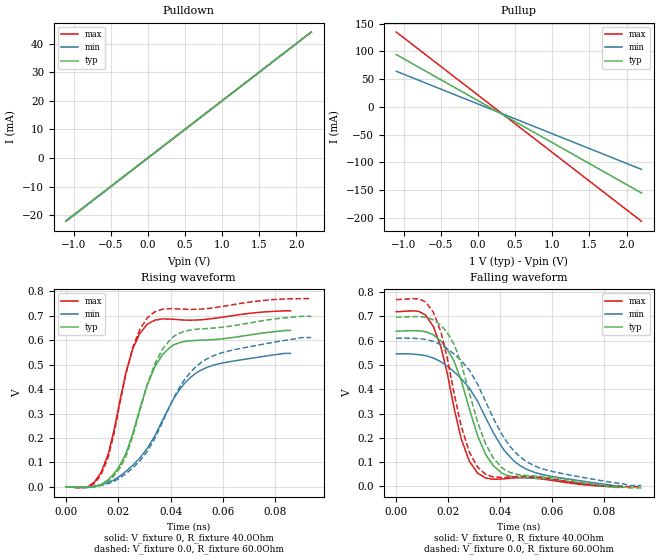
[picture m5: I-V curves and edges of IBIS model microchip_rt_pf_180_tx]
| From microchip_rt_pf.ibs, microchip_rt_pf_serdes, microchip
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|   MODEL microchip_rt_pf_180_tx
[Model] microchip_rt_pf_180_tx
Model_type   Output
Polarity   Non-Inverting
Enable   Active-High
Vmeas = 0.5
|   typ   min   max
C_comp   0.407p  0.407p  0.407p
[Voltage Range]   1.0  0.9  1.1
[Temperature Range]   60   100   0
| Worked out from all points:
|   slope of the pulldown table from 0 to 0.15 V, typ, clamps not added: 50.1 ohm
|   slope of the pullup table from 0 to 0.15 V, typ, clamps not added: 13.2 ohm
|   rising waveform, V_fixture 0, R_fixture 40.0Ohm: 20-80 % time 12.6ps typ, 19.1ps min, 9.64ps max; typ from 0 V to 0.64 V
|   rising waveform, V_fixture 0.0, R_fixture 60.0Ohm: 20-80 % time 13.3ps typ, 20ps min, 10.3ps max; typ from 0 V to 0.697 V
|   falling waveform, V_fixture 0, R_fixture 40.0Ohm: 20-80 % time 12.4ps typ, 19.3ps min, 9.67ps max; typ from 0.64 V to -0.004 V
|   falling waveform, V_fixture 0.0, R_fixture 60.0Ohm: 20-80 % time 13.2ps typ, 20.1ps min, 10.1ps max; typ from 0.697 V to -0.006 V
[Pullup]
|   X   TYP   MIN   MAX
-1.1V     94.44mA    64.32mA    135mA
1.01V     -65.12mA   -48.81mA   -83.11mA
1.089V    -71.06mA   -53.03mA   -91.23mA
2.2V      -155.1mA   -112.6mA   -206.1mA
[Pulldown]
|   X   TYP   MIN   MAX
-1.1V     -21.87mA   -22.07mA   -21.96mA
1.01V     20.25mA    20.18mA    20.22mA
1.066V    21.37mA    21.3mA     21.34mA
2.2V      44mA       44mA       44mA
[Ramp]
R_load = 50.0Ohm
|   typ   min   max
dV/dt_r   3.84E-1V/1.26E-2ns   3.27E-1V/1.91E-2ns   4.32E-1V/9.44E-3ns
dV/dt_f   3.86E-1V/1.24E-2ns   3.26E-1V/1.91E-2ns   4.33E-1V/9.31E-3ns
[Rising Waveform]
V_fixture   = 0
V_fixture_min = 0
V_fixture_max = 0
R_fixture   = 40.0Ohm
|   Time   V(typ)   V(min)   V(max)
0s        0V         0V         0V
8.626ps   -1.84mV    992.9uV    2.54mV
13.37ps   9.403mV    8.849mV    59.23mV
16.09ps   29.13mV    18.22mV    133.4mV
22.82ps   134.6mV    63.07mV    465.2mV
25.49ps   218.2mV    88.68mV    564.8mV
31.02ps   417.2mV    157.2mV    665mV
39.89ps   572mV      336.7mV    686mV
49.78ps   598.8mV    466.4mV    682.1mV
85.75ps   639.5mV    545.8mV    719.8mV
[Rising Waveform]
V_fixture   = 0.0
V_fixture_min = 0.0
V_fixture_max = 0.0
R_fixture   = 60.0Ohm
|   Time   V(typ)   V(min)   V(max)
0s        0V         0V         0V
8.626ps   -2.469mV   42.16uV    149.9uV
13.37ps   6.198mV    6.082mV    49.96mV
16.09ps   23.12mV    13.86mV    121.3mV
20.45ps   75.4mV     35.54mV    335.6mV
25.49ps   207.4mV    77.59mV    570.5mV
33.92ps   503.4mV    198.4mV    716mV
41.15ps   615.1mV    363.8mV    728.6mV
51.86ps   646mV      510.4mV    727.1mV
93.71ps   697.3mV    610.5mV    769.8mV
[Falling Waveform]
V_fixture   = 0
V_fixture_min = 0
V_fixture_max = 0
R_fixture   = 40.0Ohm
|   Time   V(typ)   V(min)   V(max)
0s        639.5mV    545.8mV    719.8mV
8.91ps    641mV      542.8mV    720.1mV
14.31ps   624.6mV    529mV      658.2mV
17.25ps   598.5mV    513.4mV    573.3mV
22.27ps   516.2mV    472.4mV    323.9mV
25.03ps   437.9mV    444.1mV    196.6mV
31.38ps   208.3mV    349.9mV    54.43mV
37.36ps   85.44mV    222.2mV    29.21mV
49.7ps    35.64mV    73.58mV    35.71mV
87.07ps   -3.979mV   1.905mV    -1.243mV
[Falling Waveform]
V_fixture   = 0.0
V_fixture_min = 0.0
V_fixture_max = 0.0
R_fixture   = 60.0Ohm
|   Time   V(typ)   V(min)   V(max)
0s        697.3mV    610.5mV    769.8mV
8.91ps    699.6mV    608.7mV    771.9mV
14.31ps   686.5mV    597.2mV    717.5mV
17.25ps   663.8mV    583.4mV    635.7mV
22.27ps   585.8mV    545.5mV    384.9mV
28.21ps   383.5mV    478.6mV    140.4mV
34.46ps   174.9mV    349.4mV    49.76mV
41.64ps   69.81mV    199.5mV    36.93mV
51.66ps   43.84mV    93.49mV    40.65mV
94.56ps   -5.988mV   3.342mV    -1.309mV
[Algorithmic Model]
Executable Linux_gcc5.4_64   MPF300T-TX_LX64.so   MPF300T-TX-R180.ami
Executable Windows_cl18.00.40629_64 MPF300T-TX_WIN64.dll  MPF300T-TX-R180.ami
Executable Windows_cl18.00.40629_32 MPF300T-TX_WIN32.dll  MPF300T-TX-R180.ami
[End Algorithmic Model]
